| IBIS file k66_180_144mbga_derated.ibs generated by Viper version: 2014.12.11
[IBIS Ver]   4.2
[Comment Char]   |_char
[File Name]   k66_180_144mbga_derated.ibs
[File Rev]   1.0
[Date]   Tue Oct 25 00:20:04 2016
[Source]   FSL Viper 2014.12.11
[Notes]
[Disclaimer] IMPORTANT NOTICE
  This information is provided on an AS IS basis and without warranty.
  IN NO EVENT SHALL Freescale BE LIABLE FOR INCIDENTAL OR CONSEQUENTIAL
  DAMAGES ARISING FROM USE OF THIS INFORMATION. THIS DISCLAIMER OF
  WARRANTY EXTENDS TO THE USER OF THE INFORMATION, AND TO THEIR CUSTOMERS
  OR USERS OF PRODUCTS  AND IS IN LIEU OF ALL WARRANTIES WHETHER EXPRESS,
  IMPLIED, OR STATUTORY, INCLUDING IMPLIED WARRANTIES OF MERCHANTABILITY
  OR FITNESS FOR PARTICULAR PURPOSE.
  Freescale does not represent or warrant that the information furnished
  hereunder is free of infringement of any third party patents,
  copyrights, trade secrets, or other intellectual property rights.
  Freescale does not represent or warrant that the information is free of
  defect, or that it meets any particular standard, requirements or need
  of the user of the infomation or their customers.
  Freescale reserves the right to change the information in this file
  without notice.
   http://www.freescale.com
[Copyright]   (C) Copyright Freescale 2004 - 2016, All Rights Reserved.
|   k66_144mbga
[Component]   k66_144mbga
[Manufacturer]   FREESCALE
[Package]
| variable   typ   min   max
R_pkg   0.13577   0.061508   0.28859
L_pkg   2.218e-9   1.085e-9   4.771e-9
C_pkg   1.168e-12   8.879e-13   2.409e-12
[Pin] signal_name   model_name   R_pin   L_pin   C_pin
A1   PTD7   p_io_fast_hd_84u3v_6m   0.18113   3.25e-9   1.512e-12
A2   PTD6   p_io_fast_hd_84u3v_6m   0.24732   3.833e-9  1.327e-12
A3   PTD5   p_io_fast_hd_84u3v_6m   0.21208   3.155e-9  1.219e-12
A4   PTD4   p_io_fast_hd_84u3v_6m   0.20624   3.081e-9  1.201e-12
A5   PTD0   p_io_fast_84u3v_6m   0.17063   2.889e-9  1.043e-12
A6   PTC16   p_io_fast_84u3v_6m   0.17309   2.843e-9  1.054e-12
A7   PTC12   p_io_fast_84u3v_6m   0.15935   2.488e-9  1.034e-12
A8   PTC8   p_io_fast_84u3v_6m   0.16032   2.635e-9  1.028e-12
A9   PTC4   p_io_fast_hd_84u3v_6m   0.13184   2.233e-9  9.86e-13
A11   PTC3   p_io_fast_hd_84u3v_6m   0.18451   2.871e-9  1.164e-12
A12   PTC2   p_io_fast_84u3v_6m   0.21085   3.32e-9   1.192e-12
B1   PTD12   p_io_fast_84u3v_6m   0.21393   3.707e-9  1.122e-12
B2   PTD11   p_io_fast_84u3v_6m   0.15724   2.583e-9  1.172e-12
B3   PTD10   p_io_fast_84u3v_6m   0.14556   2.437e-9  1.292e-12
B4   PTD3   p_io_fast_84u3v_6m   0.16088   2.48e-9   1.231e-12
B5   PTC19   p_io_fast_84u3v_6m   0.14705   2.544e-9  1.091e-12
B6   PTC15   p_io_fast_84u3v_6m   0.18502   2.732e-9  1.303e-12
B7   PTC11   p_io_fast_84u3v_6m   0.12371   2.173e-9  1.094e-12
B8   PTC7   p_io_fast_84u3v_6m   0.11477   2.073e-9  1.014e-12
B9   PTD9   p_io_fast_84u3v_6m   0.28859   4.771e-9  2.409e-12
B11   PTC1   p_io_fast_84u3v_6m   0.15501   2.628e-9  1.165e-12
B12   PTC0   p_io_fast_84u3v_6m   0.17979   3.029e-9  1.087e-12
C1   PTD15   p_io_fast_84u3v_6m   0.14879   2.588e-9  1.056e-12
C2   PTD14   p_io_fast_84u3v_6m   0.12109   2.182e-9  1.096e-12
C3   PTD13   p_io_fast_84u3v_6m   0.10733   1.981e-9  1.124e-12
C4   PTD2   p_io_fast_84u3v_6m   0.15743   2.61e-9   1.304e-12
C5   PTC18   p_io_fast_84u3v_6m   0.14372   2.436e-9  1.39e-12
C6   PTC14   p_io_fast_84u3v_6m   0.14391   2.306e-9  1.327e-12
C7   PTC10   p_io_fast_84u3v_6m   0.094596  1.85e-9   1.257e-12
C8   PTC6   p_io_fast_84u3v_6m   0.099211  1.728e-9  1.142e-12
C9   PTD8   p_io_fast_84u3v_6m   0.18207   3.12e-9   1.626e-12
C11   PTB23   p_io_fast_84u3v_6m   0.12723   2.273e-9  1.063e-12
C12   PTB22   p_io_fast_84u3v_6m   0.164   2.641e-9  1.031e-12
D1   PTE2   p_io_fast_84u3v_6m   0.15978   2.815e-9  1.026e-12
D2   PTE1   p_io_fast_84u3v_6m   0.086787  1.584e-9  1.003e-12
D3   PTE0   p_io_fast_84u3v_6m   0.083597  1.512e-9  1.042e-12
D4   PTD1   p_io_fast_84u3v_6m   0.12345   1.945e-9  1.363e-12
D5   PTC17   p_io_fast_84u3v_6m   0.11933   1.864e-9  1.409e-12
D6   PTC13   p_io_fast_84u3v_6m   0.12472   1.979e-9  1.367e-12
D7   PTC9   p_io_fast_84u3v_6m   0.11036   1.852e-9  1.345e-12
D8   PTC5   p_io_fast_84u3v_6m   0.085472  1.491e-9  1.123e-12
D9   PTB21   p_io_fast_84u3v_6m   0.072113  1.346e-9  1.135e-12
D10   PTB20   p_io_fast_84u3v_6m   0.076125  1.541e-9  1.116e-12
D11   PTB19   p_io_fast_84u3v_6m   0.12287   2.044e-9  1.066e-12
D12   PTB18   p_io_fast_84u3v_6m   0.15925   2.543e-9  1.051e-12
E1   PTE6   p_io_fast_84u3v_6m   0.15813   2.756e-9  1.046e-12
E2   PTE5   p_io_fast_84u3v_6m   0.074561  1.493e-9  9.833e-13
E3   PTE4   p_io_fast_84u3v_6m   0.15765   2.423e-9  1.315e-12
E4   PTE3   p_io_fast_84u3v_6m   0.094418  1.452e-9  1.145e-12
E5   VDD   POWER   NA   NA   NA
E6   VDD   POWER   NA   NA   NA
E7   VDD   POWER   NA   NA   NA
E8   VDD   POWER   NA   NA   NA
E9   PTB17   p_io_fast_84u3v_6m   0.092366  1.494e-9  1.16e-12
E10   PTB16   p_io_fast_84u3v_6m   0.074813  1.364e-9  1.093e-12
E11   PTB11   p_io_fast_84u3v_6m   0.12027   2.063e-9  1.006e-12
E12   PTB10   p_io_fast_84u3v_6m   0.15518   2.471e-9  1.032e-12
F1   PTE10   p_io_fast_84u3v_6m   0.15219   2.387e-9  9.957e-13
F2   PTE9   p_io_fast_84u3v_6m   0.11763   1.977e-9  1.072e-12
F3   PTE8   p_io_fast_84u3v_6m   0.15402   2.499e-9  1.272e-12
F4   PTE7   p_io_fast_84u3v_6m   0.089994  1.482e-9  1.197e-12
F5   VDD   POWER   NA   NA   NA
F6   VSS   GND   NA   NA   NA
F7   VSS   GND   NA   NA   NA
F8   VDD   POWER   NA   NA   NA
F9   PTB9   p_io_fast_84u3v_6m   0.061508  1.094e-9  1.099e-12
F10   PTB8   p_io_fast_84u3v_6m   0.073198  1.429e-9  1.067e-12
F11   PTB7   p_io_fast_84u3v_6m   0.11116   1.943e-9  9.766e-13
F12   PTB6   p_io_fast_84u3v_6m   0.14992   2.375e-9  9.927e-13
G1   VREGOUT   POWER   NA   NA   NA
G2   VREGIN0   POWER   NA   NA   NA
G3   PTE12   p_io_fast_84u3v_6m   0.078445  1.47e-9   1.206e-12
G4   PTE11   p_io_fast_84u3v_6m   0.083201  1.434e-9  1.304e-12
G5   VREFH   POWER   NA   NA   NA
G6   VREFL   NC   NA   NA   NA
G7   VSS   GND   NA   NA   NA
G8   VSS   GND   NA   NA   NA
G9   PTB5   p_io_fast_84u3v_6m   0.092341  1.466e-9  1.088e-12
G10   PTB4   p_io_fast_84u3v_6m   0.066258  1.344e-9  9.598e-13
G11   PTB3   p_io_fast_84u3v_6m   0.11636   1.826e-9  1.039e-12
G12   PTB2   p_io_fast_84u3v_6m   0.15765   2.443e-9  1.018e-12
H1   USB0DP   NC   0.18021   2.53e-9   1.161e-12
H2   USB0DM   NC   0.1724   2.42e-9   1.253e-12
H3   VSS   GND   NA   NA   NA
H4   PTE28   p_io_fast_84u3v_6m   0.13994   2.169e-9  1.679e-12
H5   VDDA   POWER   NA   NA   NA
H6   VSSA   GND   NA   NA   NA
H7   VSS   GND   NA   NA   NA
H8   VSS   GND   NA   NA   NA
H9   PTB1   p_io_fast_hd_84u3v_6m   0.090961  1.509e-9  1.122e-12
H10   PTB0   p_io_fast_hd_84u3v_6m   0.076648  1.415e-9  1.037e-12
H11   PTA29   p_io_fast_84u3v_6m   0.1127   1.984e-9  1.036e-12
H12   PTA28   p_io_fast_84u3v_6m   0.1547   2.426e-9  1.016e-12
J1   USB1DP   NC   0.16139   2.181e-9  1.017e-12
J2   VREGIN1   POWER   NA   NA   NA
J3   ADC0SE16_CMP1IN2_ADC0SE21   NC   0.095501  1.904e-9  1.256e-12
J4   PTE27   p_io_fast_84u3v_6m   0.13441   2.201e-9  1.755e-12
J5   PTA0   p_io_fast_84u3v_6m   0.15672   2.486e-9  1.406e-12
J6   PTA1   p_io_fast_84u3v_6m   0.13639   2.166e-9  1.409e-12
J7   PTA6   p_io_fast_84u3v_6m   0.06478   1.085e-9  1.126e-12
J8   PTA7   p_io_fast_84u3v_6m   0.086884  1.412e-9  1.25e-12
J9   PTA13   p_io_fast_84u3v_6m   0.07931   1.389e-9  1.179e-12
J10   PTA27   p_io_fast_84u3v_6m   0.064689  1.279e-9  1.148e-12
J11   PTA26   p_io_fast_84u3v_6m   0.11469   1.919e-9  9.807e-13
J12   PTA25   p_io_fast_84u3v_6m   0.15109   2.38e-9   9.914e-13
K1   USB1DM   NC   0.1573   2.132e-9  9.936e-13
K2   VSS   GND   NA   NA   NA
K3   ADC1SE16_CMP2IN2_ADC0SE22   NC   0.094276  1.753e-9  1.032e-12
K4   PTE26   p_io_fast_84u3v_6m   0.11922   2.143e-9  1.713e-12
K5   PTE25   p_io_fast_84u3v_6m   0.075131  1.394e-9  1.793e-12
K6   PTA2   p_io_fast_84u3v_6m   0.074132  1.541e-9  1.124e-12
K7   PTA3   p_io_fast_84u3v_6m   0.078318  1.485e-9  9.801e-13
K8   PTA8   p_io_fast_84u3v_6m   0.1672   2.519e-9  1.304e-12
K9   PTA12   p_io_fast_84u3v_6m   0.0801   1.495e-9  1.118e-12
K10   PTA16   p_io_fast_84u3v_6m   0.12824   2.015e-9  1.235e-12
K11   PTA17   p_io_fast_84u3v_6m   0.14899   2.329e-9  1.281e-12
K12   PTA24   p_io_fast_84u3v_6m   0.12452   2.165e-9  9.714e-13
L1   USB1VBUS   POWER   NA   NA   NA
L2   ADC0DM0_ADC1DM3   NC   0.18768   2.585e-9  1.149e-12
L3   DAC0OUT_CMP1IN3_ADC0SE23   NC   0.12476   1.908e-9  9.444e-13
L4   DAC1OUT_CMP0IN4_CMP2IN3_ADC1SE23   NC   0.11527   2.047e-9  9.975e-13
L5   TAMPER0   p_io_84u3v_6m   0.12498   2.023e-9  1.1e-12
L6   VBAT   POWER   NA   NA   NA
L7   PTA4   p_io_flt_84u3v_6m   0.11749   1.933e-9  1.001e-12
L8   PTA9   p_io_fast_84u3v_6m   0.11363   1.868e-9  1.037e-12
L9   PTA11   p_io_fast_84u3v_6m   0.12841   2.094e-9  1.096e-12
L10   PTA14   p_io_fast_84u3v_6m   0.14575   2.167e-9  1.114e-12
L11   PTA15   p_io_fast_84u3v_6m   0.15617   2.398e-9  1.109e-12
L12   RESETB   p_vpp_84u3v_6m   0.12233   2.294e-9  1.078e-12
M1   ADC1DP0_ADC0DP3   NC   0.22522   3.192e-9  1.336e-12
M2   ADC1DM0_ADC0DM3   NC   0.23133   3.286e-9  1.261e-12
M3   VREFOUT_CMP1IN5_CMP0IN5_ADC1SE18   NC   NA   NA   NA
M4   PTE24   p_io_fast_84u3v_6m   0.19026   2.885e-9  1.138e-12
M6   EXTAL32   NC   0.13628   2.197e-9  8.879e-13
M7   XTAL32   NC   0.19201   2.999e-9  1.094e-12
M8   PTA5   p_io_fast_84u3v_6m   0.17055   2.428e-9  1.044e-12
M9   PTA10   p_io_fast_84u3v_6m   0.16425   2.473e-9  1.009e-12
M10   VSS   GND   NA   NA   NA
M11   PTA19   p_io_fast_84u3v_6m   0.21399   3.114e-9  1.185e-12
M12   PTA18   p_io_fast_84u3v_6m   0.1793   2.688e-9  1.102e-12
[Pin Mapping]   pulldown_ref   pullup_ref
A1   NC   NC
A2   NC   NC
A3   NC   NC
A4   NC   NC
A5   NC   NC
A6   NC   NC
A7   NC   NC
A8   NC   NC
A9   NC   NC
A11   NC   NC
A12   NC   NC
B1   NC   NC
B2   NC   NC
B3   NC   NC
B4   NC   NC
B5   NC   NC
B6   NC   NC
B7   NC   NC
B8   NC   NC
B9   NC   NC
B11   NC   NC
B12   NC   NC
C1   NC   NC
C2   NC   NC
C3   NC   NC
C4   NC   NC
C5   NC   NC
C6   NC   NC
C7   NC   NC
C8   NC   NC
C9   NC   NC
C11   NC   NC
C12   NC   NC
D1   NC   NC
D2   NC   NC
D3   NC   NC
D4   NC   NC
D5   NC   NC
D6   NC   NC
D7   NC   NC
D8   NC   NC
D9   NC   NC
D10   NC   NC
D11   NC   NC
D12   NC   NC
E1   NC   NC
E2   NC   NC
E3   NC   NC
E4   NC   NC
E5   NC   VDD
E6   NC   VDD
E7   NC   VDD
E8   NC   VDD
E9   NC   NC
E10   NC   NC
E11   NC   NC
E12   NC   NC
F1   NC   NC
F2   NC   NC
F3   NC   NC
F4   NC   NC
F5   NC   VDD
F6   VSS   NC
F7   VSS   NC
F8   NC   VDD
F9   NC   NC
F10   NC   NC
F11   NC   NC
F12   NC   NC
G1   NC   VREGOUT
G2   NC   VREGIN0
G3   NC   NC
G4   NC   NC
G5   NC   VREFH
G6   NC   NC
G7   VSS   NC
G8   VSS   NC
G9   NC   NC
G10   NC   NC
G11   NC   NC
G12   NC   NC
H1   NC   NC
H2   NC   NC
H3   VSS   NC
H4   NC   NC
H5   NC   VDDA
H6   VSSA   NC
H7   VSS   NC
H8   VSS   NC
H9   NC   NC
H10   NC   NC
H11   NC   NC
H12   NC   NC
J1   NC   NC
J2   NC   VREGIN1
J3   NC   NC
J4   NC   NC
J5   NC   NC
J6   NC   NC
J7   NC   NC
J8   NC   NC
J9   NC   NC
J10   NC   NC
J11   NC   NC
J12   NC   NC
K1   NC   NC
K2   VSS   NC
K3   NC   NC
K4   NC   NC
K5   NC   NC
K6   NC   NC
K7   NC   NC
K8   NC   NC
K9   NC   NC
K10   NC   NC
K11   NC   NC
K12   NC   NC
L1   NC   USB1VBUS
L2   NC   NC
L3   NC   NC
L4   NC   NC
L5   NC   NC
L6   NC   VBAT
L7   NC   NC
L8   NC   NC
L9   NC   NC
L10   NC   NC
L11   NC   NC
L12   NC   NC
M1   NC   NC
M2   NC   NC
M3   NC   NC
M4   NC   NC
M6   NC   NC
M7   NC   NC
M8   NC   NC
M9   NC   NC
M10   VSS   NC
M11   NC   NC
M12   NC   NC
|*   Model Selector   *
[Model Selector] p_io_84u3v_6m
p_io_84u3v_6m_sre0   io, without slew rate
p_io_84u3v_6m_sre1   io, with slew rate
[Model Selector] p_io_fast_84u3v_6m
p_io_fast_84u3v_6m_sre0   io, without slew rate
p_io_fast_84u3v_6m_sre1   io, with slew rate
[Model Selector] p_io_fast_hd_84u3v_6m
p_io_fast_hd_84u3v_6m_obe1dse0sre0   io 5mA, without slew rate
p_io_fast_hd_84u3v_6m_obe1dse0sre1   io 5mA, with slew rate
p_io_fast_hd_84u3v_6m_obe1dse1sre0   io 20mA, without slew rate
p_io_fast_hd_84u3v_6m_obe1dse1sre1   io 20mA, with slew rate
[Model Selector] p_io_flt_84u3v_6m
p_io_flt_84u3v_6m_sre0   io_flt, without slew rate
p_io_flt_84u3v_6m_sre1   io_flt, with slew rate
| End [Component] k66_144mbga
| Models and submodels in the file (11): p_io_84u3v_6m_sre0 (I/O), p_io_84u3v_6m_sre1 (I/O), p_io_fast_84u3v_6m_sre0 (I/O), p_io_fast_84u3v_6m_sre1 (I/O), p_io_fast_hd_84u3v_6m_obe1dse0sre0 (I/O), p_io_fast_hd_84u3v_6m_obe1dse0sre1 (I/O), p_io_fast_hd_84u3v_6m_obe1dse1sre0 (I/O), p_io_fast_hd_84u3v_6m_obe1dse1sre1 (I/O), p_io_flt_84u3v_6m_sre0 (I/O), p_io_flt_84u3v_6m_sre1 (I/O), p_vpp_84u3v_6m (I/O_open_drain)
